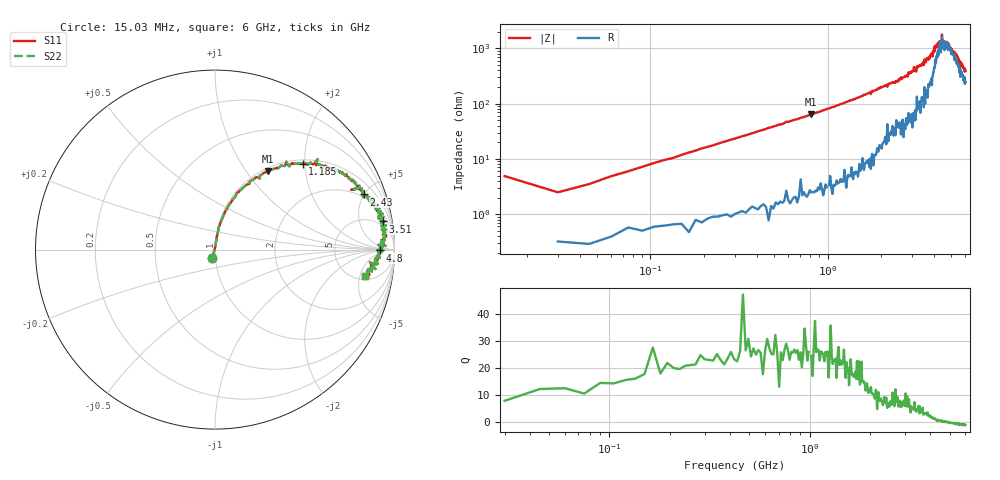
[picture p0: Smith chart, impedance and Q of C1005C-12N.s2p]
!	Network	Analyzer	HP8753E.07.74:	Oct	30	2002	Serial	No.	JP38451487
!	Hewlett-Packard
!	7	Sep	2009	8:43:02
!	Frequency	S11	S21	S12	S22
#	HZ	S	RI	R	50
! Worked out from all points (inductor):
!   400 points, 15.03 MHz to 6 GHz, reference 50 ohm
!   read as one part in series: L = 12.6 nH near 45.03 MHz
!   highest Q = 26.5 at 810 MHz (marker M1), where L = 12.5 nH
!   self-resonance near 4.598 GHz
!   S11 on the Smith chart (normalised r, x): 15.03 MHz: 0.97, -0.09; 1.185 GHz: 1.09, +1.95; 2.43 GHz: 1.77, +4.97; 3.51 GHz: 4, +11; 4.8 GHz: 23, -1; 6 GHz: 5.85, -6.14
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1.502992e7  -0.0148 -0.048  1.01 0.048  1.01 0.048  -0.0148 -0.048
3.002985e7  0.0036 0.0245  0.996 -0.0245  0.996 -0.0245  0.0036 0.0245
1.050295e8  0.0127 0.0827  0.987 -0.0827  0.987 -0.0827  0.0127 0.0827
2.550287e8  0.0469 0.189  0.953 -0.189  0.953 -0.189  0.0469 0.189
8.10026e8  0.297 0.438  0.703 -0.438  0.703 -0.438  0.297 0.438
1.020025e9  0.406 0.471  0.594 -0.471  0.594 -0.471  0.406 0.471
1.185024e9  0.488 0.478  0.512 -0.478  0.512 -0.478  0.488 0.478
2.01002e9  0.774 0.376  0.226 -0.376  0.226 -0.376  0.774 0.376
2.430018e9  0.829 0.307  0.171 -0.307  0.171 -0.307  0.829 0.307
3.015015e9  0.918 0.23  0.0817 -0.23  0.0817 -0.23  0.918 0.23
3.510012e9  0.935 0.157  0.0652 -0.157  0.0652 -0.157  0.935 0.157
3.91501e9  0.929 0.111  0.0708 -0.111  0.0708 -0.111  0.929 0.111
4.00501e9  0.955 0.078  0.0446 -0.078  0.0446 -0.078  0.955 0.078
4.335008e9  0.932 0.0158  0.0676 -0.0158  0.0676 -0.0158  0.932 0.0158
4.365008e9  0.926 0.0487  0.0739 -0.0487  0.0739 -0.0487  0.926 0.0487
4.425008e9  0.951 0.02  0.0495 -0.02  0.0495 -0.02  0.951 0.02
4.455008e9  0.919 0.0279  0.0808 -0.0279  0.0808 -0.0279  0.919 0.0279
4.485008e9  0.936 0.0185  0.0642 -0.0185  0.0642 -0.0185  0.936 0.0185
4.575007e9  0.911 0.0267  0.0892 -0.0267  0.0892 -0.0267  0.911 0.0267
4.800006e9  0.918 -0.00482  0.0823 0.00482  0.0823 0.00482  0.918 -0.00482
5.010005e9  0.909 -0.0312  0.0906 0.0312  0.0906 0.0312  0.909 -0.0312
6e9  0.838 -0.145  0.162 0.145  0.162 0.145  0.838 -0.145
